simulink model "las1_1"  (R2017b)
settings: Solver=ode45  StartTime=0.0  StopTime=300  MaxStep=1  RelTol=1e-3  AbsTol=1e-3
libraries: simulink x1

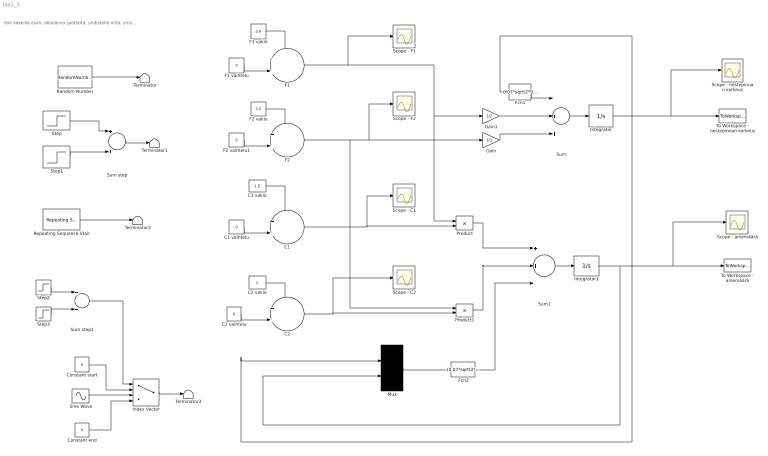
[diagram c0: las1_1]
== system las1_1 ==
  note: Voit kokeilla esim. allaolevia syötteitä, yhdistellä niitä, yms...
  C1 : Sum  Inputs=++|
  C1 vaihtelu : Constant  Value=0
  C1 vakio : Constant  Value=1.5
  C2 : Sum  Inputs=++|
  C2 vaihtelu : Constant  Value=0
  C2 vakio : Constant
  Constant end : Constant  Value=0
  Constant start : Constant  Value=0
  F1 : Sum  Inputs=++|
  F1 vaihtelu : Constant  Value=0
  F1 vakio : Constant  Value=0.9
  F2 : Sum  Inputs=++|
  F2 vaihtelu1 : Constant  Value=0
  F2 vakio : Constant  Value=0.3
  Fcn1 : Fcn  Expr=0.07*sqrt(2*9.81*u)/2
  Fcn2 : Fcn  Expr=(0.07*sqrt(2*9.81)*u[2])/(2*sqrt(u[1]))
  Gain : Gain  Gain=1/2
  Gain1 : Gain  Gain=1/2
  Index Vector : MultiPortSwitch  DataPortOrder=Zero-based contiguous  zeroidx=on
  Integrator : Integrator  InitialCondition=1.5
  Integrator1 : Integrator  InitialCondition=10
  Mux : Mux  Inputs=2
  Product : Product
  Product1 : Product
  Random Number : RandomNumber  Variance=0.05  SampleTime=0.1
  Repeating Sequence Stair : simulink/Sources/Repeating Sequence Stair  OutValues=[0.2 0 0.2 0].'  tsamp=50  OutMin=[]  OutMax=[]  OutDataTypeStr=double  OutputDataTypeScalingMode=Specify via dialog  OutDataType=double  ConRadixGroup=Best Precision: Vector-wise  OutScaling=2^-12
  Scope - ainemäärä : Scope
  Scope - nestepinnan korkeus : Scope
  Scope - C1 : Scope
  Scope - C2 : Scope
  Scope - F1 : Scope
  Scope - F2 : Scope
  Sine Wave : Sin  Amplitude=0.2  Frequency=0.1  Phase=1  SampleTime=0.1
  Step : Step  Time=25  SampleTime=0
  Step1 : Step  Time=50  After=-1  SampleTime=0
  Step2 : Step  Time=25  SampleTime=0
  Step3 : Step  Time=100  SampleTime=0
  Sum : Sum  Inputs=-++
  Sum step : Sum
  Sum step1 : Sum
  Sum1 : Sum  Inputs=++-
  Terminator{,1..3} (4 alike) : Terminator
  To Workspace - ainemäärä : ToWorkspace  VariableName=n
  To Workspace - nestepinnan korkeus : ToWorkspace  VariableName=h
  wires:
  Mux/1 -> Fcn2/1
  Integrator/1 -> To Workspace - nestepinnan korkeus/1, Scope - nestepinnan korkeus/1, Mux/1, Fcn1/1
  Product1/1 -> Sum1/2
  Product/1 -> Sum1/1
  Sum1/1 -> Integrator1/1
  F2/1 -> Gain/1, Scope - F2/1, Product1/1
  F1/1 -> Scope - F1/1, Product/1, Gain1/1
  F1 vakio/1 -> F1/1
  Fcn1/1 -> Sum/1
  F2 vakio/1 -> F2/1
  C1/1 -> Product/2, Scope - C1/1
  C1 vakio/1 -> C1/1
  C2/1 -> Product1/2, Scope - C2/1
  C2 vakio/1 -> C2/1
  Fcn2/1 -> Sum1/3
  Integrator1/1 -> Mux/2, To Workspace - ainemäärä/1, Scope - ainemäärä/1
  Step1/1 -> Sum step/2
  Step/1 -> Sum step/1
  Random Number/1 -> Terminator/1
  Sum step/1 -> Terminator1/1
  Repeating Sequence Stair/1 -> Terminator2/1
  Sine Wave/1 -> Index Vector/3
  Constant end/1 -> Index Vector/4
  Constant start/1 -> Index Vector/2
  Step2/1 -> Sum step1/1
  Step3/1 -> Sum step1/2
  Sum step1/1 -> Index Vector/1
  Index Vector/1 -> Terminator3/1
  F2 vaihtelu1/1 -> F2/2
  C2 vaihtelu/1 -> C2/2
  C1 vaihtelu/1 -> C1/2
  F1 vaihtelu/1 -> F1/2
  Sum/1 -> Integrator/1
  Gain1/1 -> Sum/2
  Gain/1 -> Sum/3
